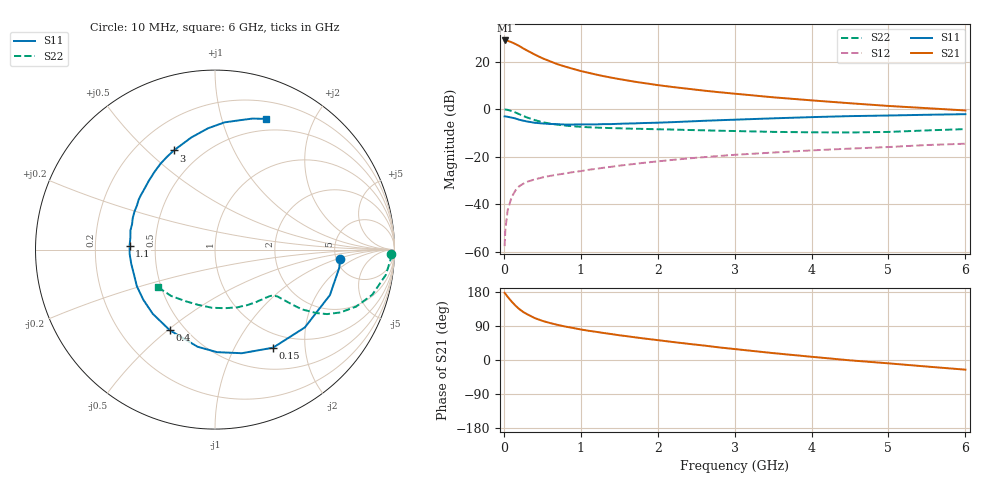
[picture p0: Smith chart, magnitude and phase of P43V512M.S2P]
! SIEMENS Small Signal Semiconductors
! BFP182
! Si NPN RF Bipolar Junction Transistor in SOT143
! VCE = 3.5 V  IC = 12 mA
! Common Emitter S-Parameters:  March  1996
# GHz  S  MA  R  50
!  f  S11  S21  S12  S22
! GHz  MAG  ANG  MAG  ANG  MAG  ANG  MAG  ANG
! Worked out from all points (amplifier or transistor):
!   36 points, 10 MHz to 6 GHz, reference 50 ohm
!   highest |S21| = 28.9 dB at 20 MHz (marker M1)
!   |S21| within 3 dB of that: start of sweep to 234.7 MHz
!   unconditionally stable (mu >= 1): 1.069 GHz to 5.392 GHz
!   at 250 MHz: K = 0.37, MSG = 28.5 dB, |S12| = -31.5 dB
!   at 1.4 GHz: K = 1.10, MAG = 16.8 dB, |S12| = -24.3 dB
!   at 6 GHz: K = 0.93, MSG = 7.0 dB, |S12| = -14.6 dB
!   S11 on the Smith chart (normalised r, x): 10 MHz: 5.46, -1.07; 150 MHz: 0.79, -1.44; 400 MHz: 0.42, -0.51; 1.1 GHz: 0.35, +0.02; 3 GHz: 0.35, +0.61; 6 GHz: 0.37, +1.40
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0.01  0.7004 -4.1  27.83 177.2  0.0013 84.6  0.9784 -1.5
0.02  0.6997 -8.4  27.84 174.9  0.0029 85.0  0.9796 -3.3
0.05  0.6886 -21.6  27.42 166.7  0.0075 82.9  0.9621 -8.4
0.1  0.6623 -40.9  25.6 154.5  0.0138 70.5  0.9118 -16.0
0.15  0.635 -59.4  23.49 143.7  0.0193 63.9  0.848 -22.0
0.2  0.5963 -75.5  21.33 134.5  0.0238 58.8  0.7816 -26.6
0.25  0.5715 -88.9  19.04 127.0  0.0267 54.3  0.7209 -29.9
0.3  0.5497 -100.2  17.19 121.1  0.0294 51.5  0.6676 -32.0
0.4  0.5152 -119.2  14.11 110.8  0.033 48.7  0.5883 -34.5
0.5  0.4982 -134.2  11.77 103.4  0.0363 46.3  0.5317 -35.4
0.6  0.4873 -145.1  10.15 97.6  0.0392 45.8  0.4942 -35.9
0.7  0.4809 -154.9  8.779 92.6  0.0418 46.1  0.4685 -36.3
0.9  0.4733 -170.3  7.02 84.5  0.0471 46.4  0.4348 -36.9
1.1  0.4763 177.4  5.809 77.2  0.0526 47.0  0.4148 -38.3
1.5  0.4906 159.2  4.283 65.3  0.0644 47.4  0.3942 -42.2
1.8  0.5079 147.0  3.57 57.4  0.0733 46.9  0.3832 -46.3
2.2  0.5312 134.1  2.908 47.4  0.0854 45.1  0.3708 -52.7
3  0.5982 112.5  2.111 28.9  0.1089 39.7  0.3453 -68.6
3.5  0.6383 102.0  1.771 18.2  0.1216 35.8  0.3313 -80.3
4.5  0.7109 85.7  1.327 -0.9  0.1472 28.1  0.3218 -106.8
5.5  0.7589 74.1  1.045 -17.3  0.1751 20.5  0.3557 -133.5
6  0.7818 68.7  0.935 -25.5  0.1867 15.8  0.3793 -146.2
